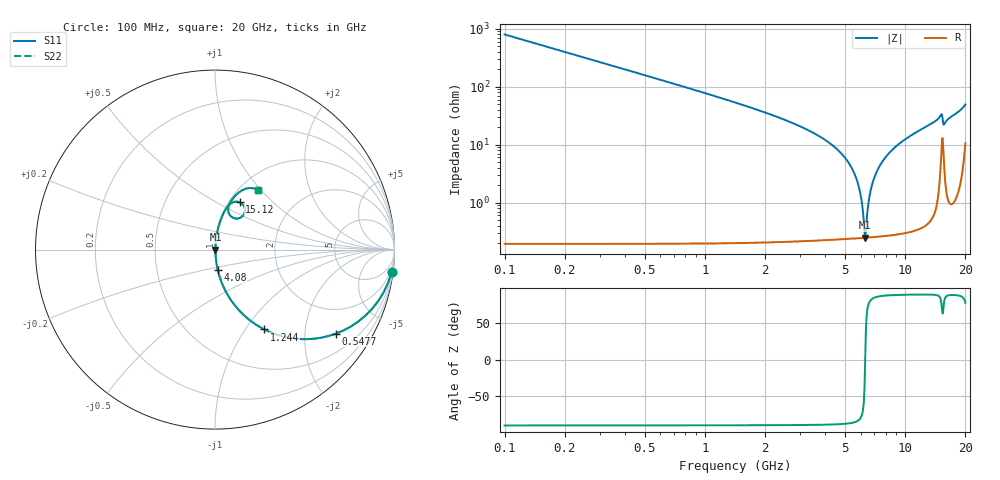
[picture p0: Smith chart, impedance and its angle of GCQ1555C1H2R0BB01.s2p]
!Murata Part Number: GCQ1555C1H2R0BB01
!These Parameters are Measured in Series Mode Connection
!Data Generated on Mar 13, 2026
!  o--ll--o
!Port1  Port2
!  o------o
!Operation Temp=25[degC], DC Bias Voltage=0[V]
!Freq. Start=100[MHz] Stop=20[GHz] 401[Steps]
# Hz S RI R 50
!Freq.(Hz) S11(Real) S11(Imag) S21(Real) S21(Imag) S12(Real) S12(Imag) S22(Real) S22(Imag)
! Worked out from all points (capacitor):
!   401 points, 100 MHz to 20 GHz, reference 50 ohm
!   read as one part in series: C = 2 pF near 199.5 MHz
!   lowest |Z| = 247 mohm at 6.319 GHz (marker M1)
!   series resonance near 6.319 GHz, so ESL is about 320 pH
!   S11 on the Smith chart (normalised r, x): 100 MHz: 1, -16; 547.8 MHz: 1.00, -2.88; 1.244 GHz: 1.00, -1.23; 4.08 GHz: 1.00, -0.23; 15.12 GHz: 1.12, +0.65; 20 GHz: 1.21, +0.96
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1e8  0.9844 -0.1237  0.0156 0.1237  0.0156 0.1237  0.9844 -0.1237
2.99e8  0.8756 -0.3296  0.1244 0.3296  0.1244 0.3296  0.8756 -0.3296
5.4775e8  0.675 -0.4677  0.325 0.4677  0.325 0.4677  0.675 -0.4677
1.24425e9  0.275 -0.4449  0.725 0.4449  0.725 0.4449  0.275 -0.4449
2.09e9  0.1047 -0.3032  0.8953 0.3032  0.8953 0.3032  0.1047 -0.3032
3.43325e9  0.0281 -0.1587  0.9719 0.1587  0.9719 0.1587  0.0281 -0.1587
4.08e9  0.015 -0.1121  0.985 0.1121  0.985 0.1121  0.015 -0.1121
5.02525e9  0.00573 -0.058  0.9943 0.058  0.9943 0.058  0.00573 -0.058
5.62225e9  0.00327 -0.0295  0.9967 0.0295  0.9967 0.0295  0.00327 -0.0295
5.9705e9  0.00264 -0.0143  0.9974 0.0143  0.9974 0.0143  0.00264 -0.0143
6.21925e9  0.00247 -0.00401  0.9975 0.00401  0.9975 0.00401  0.00247 -0.00401
6.31875e9  0.00247 2.5e-06  0.9975 -2.5e-06  0.9975 -2.5e-06  0.00247 2.5e-06
6.61725e9  0.00263 0.0117  0.9974 -0.0117  0.9974 -0.0117  0.00263 0.0117
6.7665e9  0.00281 0.0173  0.9972 -0.0173  0.9972 -0.0173  0.00281 0.0173
7.21425e9  0.0037 0.0337  0.9963 -0.0337  0.9963 -0.0337  0.0037 0.0337
7.861e9  0.00577 0.0558  0.9942 -0.0558  0.9942 -0.0558  0.00577 0.0558
1.005e10  0.0182 0.1221  0.9818 -0.1221  0.9818 -0.1221  0.0182 0.1221
1.338325e10  0.0523 0.2122  0.9477 -0.2122  0.9477 -0.2122  0.0523 0.2122
1.51245e10  0.137 0.2641  0.863 -0.2641  0.863 -0.2641  0.137 0.2641
1.557225e10  0.0956 0.18  0.9044 -0.18  0.9044 -0.18  0.0956 0.18
1.67165e10  0.0855 0.2636  0.9145 -0.2636  0.9145 -0.2636  0.0855 0.2636
2e10  0.2398 0.3309  0.7602 -0.3309  0.7602 -0.3309  0.2398 0.3309
